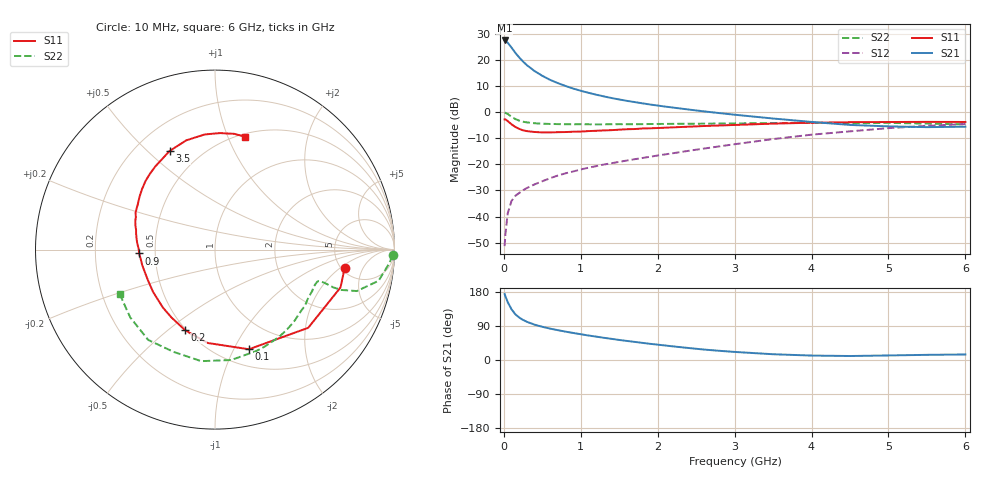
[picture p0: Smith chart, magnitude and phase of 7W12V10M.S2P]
! Infineon Technologies  Discrete & RF Semiconductors
! BFS17W
! Si NPN RF Bipolar Junction Transistor in SOT323
! VCE = 12 V  IC = 10 mA
! Common Emitter S-Parameters:  August  1999
# GHz  S  MA  R  50
!  f  S11  S21  S12  S22
! GHz  MAG  ANG  MAG  ANG  MAG  ANG  MAG  ANG
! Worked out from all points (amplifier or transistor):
!   36 points, 10 MHz to 6 GHz, reference 50 ohm
!   highest |S21| = 27.5 dB at 10 MHz (marker M1)
!   |S21| within 3 dB of that: start of sweep to 106.4 MHz
!   unconditionally stable (mu >= 1): 455 MHz to 2.098 GHz; 5.708 GHz to end of sweep
!   at 250 MHz: K = 0.75, MSG = 24.7 dB, |S12| = -29.9 dB
!   at 1.4 GHz: K = 1.15, MAG = 10.1 dB, |S12| = -19.6 dB
!   at 6 GHz: K = 1.02, MAG = -1.4 dB, |S12| = -4.5 dB
!   S11 on the Smith chart (normalised r, x): 10 MHz: 5.31, -2.36; 100 MHz: 0.68, -1.15; 200 MHz: 0.49, -0.58; 900 MHz: 0.41, -0.02; 3.5 GHz: 0.34, +0.59; 6 GHz: 0.53, +1.16
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0.01  0.7295 -8.2  23.82 174.2  0.0027 78.1  0.9906 -1.9
0.02  0.7303 -16.8  23.52 168.3  0.0045 88.0  0.9723 -4.7
0.05  0.6779 -40.0  21.61 152.9  0.0115 73.0  0.9278 -10.8
0.1  0.5865 -71.2  17.37 133.7  0.0199 62.3  0.8232 -16.3
0.15  0.5219 -94.5  13.8 120.6  0.025 57.1  0.7396 -17.7
0.2  0.4793 -110.2  11.23 112.0  0.0283 56.3  0.6899 -17.7
0.25  0.4497 -122.5  9.351 105.7  0.0319 55.5  0.6583 -17.2
0.3  0.4344 -131.9  7.988 100.8  0.0353 57.4  0.6382 -16.9
0.4  0.4179 -145.7  6.158 93.2  0.0414 59.0  0.6148 -16.7
0.5  0.4109 -155.1  4.997 87.6  0.0475 61.6  0.6031 -16.9
0.6  0.4107 -162.2  4.189 82.9  0.0542 63.3  0.5963 -17.5
0.7  0.4146 -168.0  3.628 78.8  0.061 65.5  0.5924 -18.7
0.9  0.4229 -177.1  2.85 71.4  0.073 67.5  0.5868 -21.4
1.1  0.435 175.2  2.36 64.6  0.0864 68.4  0.5866 -24.8
1.3  0.4484 168.6  2.014 58.6  0.0994 69.8  0.5856 -28.6
1.6  0.4723 160.1  1.653 50.3  0.1186 71.0  0.5889 -34.6
2.2  0.5133 145.0  1.228 35.9  0.1638 73.8  0.5992 -48.1
2.8  0.5573 130.4  0.964 24.3  0.2214 73.8  0.6074 -63.1
3.5  0.605 114.7  0.758 15.2  0.3058 70.3  0.6218 -81.7
4.5  0.6441 95.1  0.571 10.5  0.43 58.9  0.6148 -112.0
5.5  0.6538 80.6  0.518 13.6  0.5476 45.6  0.6047 -141.4
6  0.651 74.9  0.528 14.6  0.5946 38.8  0.5858 -154.8
